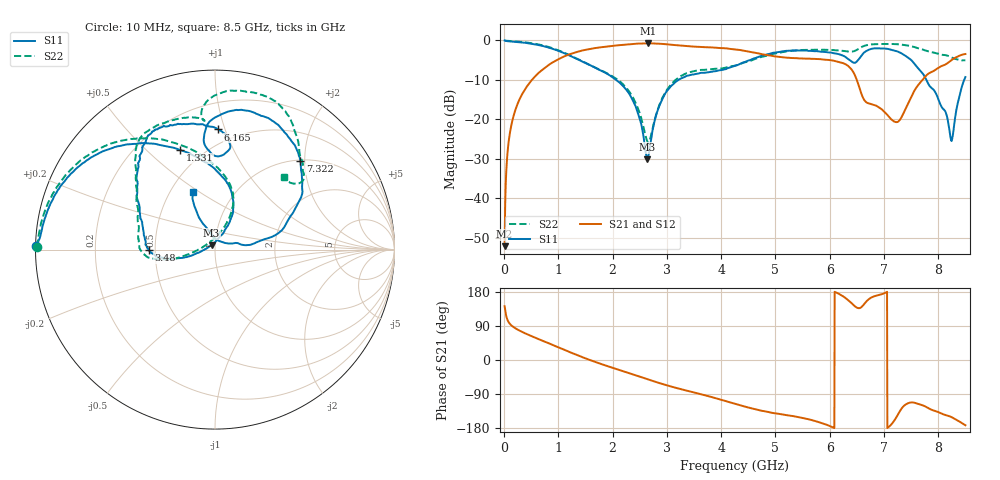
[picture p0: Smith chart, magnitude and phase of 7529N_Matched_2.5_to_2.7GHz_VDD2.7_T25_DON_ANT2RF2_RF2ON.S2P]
!Agilent Technologies,E5071C,MY46417908,A.11.23
!Date: Wed Oct 16 15:59:14 2019
!Data & Calibration Information:
!Freq	S11:SOLT2(ON)	S21:SOLT2(ON)	S12:SOLT2(ON)	S22:SOLT2(ON)
!PortZ  Port1:50+j0  Port2:50+j0
!Above PortZ is port z conversion or system Z0 setting when saving the data.
!When reading, reference impedance value at option line is always used.
# Hz S dB R 50
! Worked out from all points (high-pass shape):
!   1601 points, 10 MHz to 8.5 GHz, reference 50 ohm
!   highest |S21| = -0.73 dB at 2.653 GHz (marker M1); lowest = -52.2 dB at 10 MHz (marker M2)
!   |S21| within 3 dB of the highest: 1.167 GHz to 4.861 GHz (3.694 GHz wide, 123 % of centre); 8.418 GHz to end of sweep
!   lowest |S11| = -30.1 dB at 2.642 GHz (marker M3), VSWR 1.06, Z = 48.1 + j2.37 ohm
!   |S11| at or under -10 dB: 2.066 GHz to 3.216 GHz (1.151 GHz wide, 43.6 % of centre); 7.781 GHz to 8.479 GHz (698 MHz wide, 8.59 % of centre)
!   |S22| runs from -25.8 to -0.1 dB; largest |S21 - S12| = 0.0071
!   S11 on the Smith chart (normalised r, x): 10 MHz: 0.00, +0.01; 1.331 GHz: 0.38, +0.64; 3.48 GHz: 0.46, -0.00; 6.165 GHz: 0.39, +0.95; 7.322 GHz: 1.02, +1.91; 8.5 GHz: 0.65, +0.47
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1e7  -0.02 178.9  -52.17 142.0  -52.13 141.7  -0.06 179.1
9.49e7  -0.24 174.2  -24.64 97.6  -24.66 97.7  -0.14 174.4
2.700062e8  -0.43 164.8  -15.39 78.7  -15.44 78.7  -0.29 164.5
8.1655e8  -1.81 136.4  -6.29 44.6  -6.33 44.8  -1.65 134.4
1.331256e9  -4.61 109.2  -2.97 13.9  -3.00 14.1  -4.54 105.6
1.426769e9  -5.26 104.0  -2.61 8.5  -2.63 8.6  -5.20 100.3
2.281075e9  -13.03 63.7  -1.02 -33.5  -1.03 -33.5  -12.52 66.9
2.477406e9  -18.91 62.9  -0.81 -42.7  -0.82 -42.7  -17.65 68.3
2.6419e9  -30.14 127.6  -0.74 -50.6  -0.74 -50.6  -25.68 117.3
2.652512e9  -29.61 140.6  -0.73 -51.1  -0.73 -51.1  -25.77 125.8
2.843538e9  -17.23 -165.6  -0.83 -60.0  -0.82 -60.1  -17.03 -171.1
3.480288e9  -8.63 -179.7  -1.56 -84.9  -1.56 -85.0  -7.87 -177.6
4.255e9  -6.47 152.3  -2.30 -115.2  -2.32 -115.4  -6.41 153.5
5.671769e9  -2.67 109.4  -4.69 -158.7  -4.64 -158.6  -2.38 117.6
6.16525e9  -3.48 88.4  -5.46 175.0  -5.44 174.9  -2.54 99.4
6.446481e9  -5.68 87.6  -8.33 144.0  -8.36 144.1  -2.74 95.4
6.605669e9  -3.49 94.6  -14.31 142.6  -14.35 142.6  -1.56 92.5
7.088538e9  -2.23 62.2  -19.33 -176.7  -19.40 -176.8  -0.91 73.8
7.322012e9  -3.28 46.0  -19.52 -128.5  -19.56 -128.7  -1.05 66.7
7.937538e9  -12.98 9.2  -7.57 -134.2  -7.56 -134.4  -3.17 46.0
8.239994e9  -25.42 61.6  -5.04 -150.5  -4.99 -150.4  -4.30 38.0
8.5e9  -9.30 111.3  -3.45 -172.2  -3.41 -172.2  -5.03 46.5
